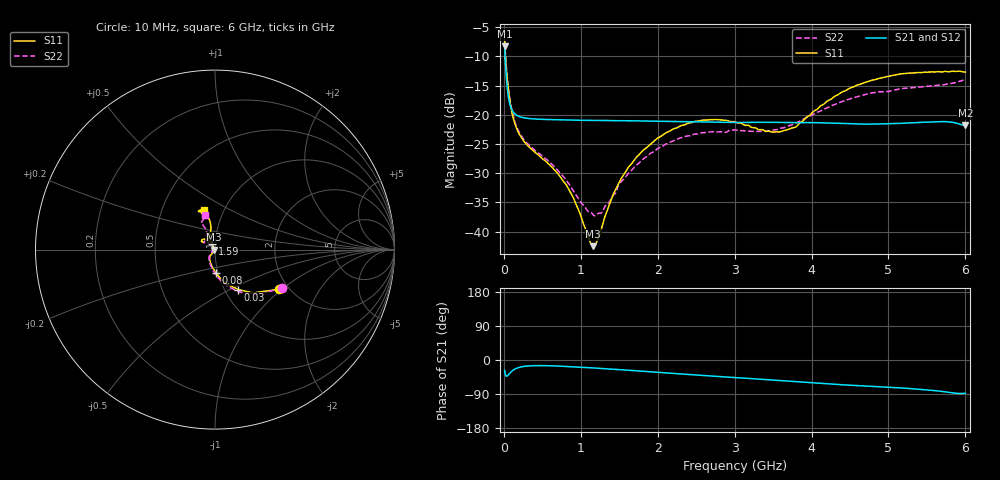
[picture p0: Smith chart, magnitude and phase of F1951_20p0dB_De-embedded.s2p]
! Integrated Device Technology
! Corporate Headquarters
! 6024 Silver Creek Valley Road
! San Jose, CA 95138  USA
! Phone:  1-408-284-8200
! Toll Free:  1-800-223-1366
! Webpage:  http://www.idt.com/
! Timing and RF Division
! 515 Groton Road, Suite 102
! Westford, MA 01886-6024
! Device:  F1951
! Description: 6-bit 0.5 dB Digital Step Attenuator
! Frequency:  100.0 -  4000.00 MHz
! Package:  4x4 mm Thin QFN Plastic Package: 24 pin
! Ports:  2 RF, 6 DC
!  Pin  1  = NC
!  Pin  2  = RF1  =  Port 1
!  Pin  3  = GND
!  Pin  4  = NC
!  Pin  5  = Serial Data Out (SDO)
!  Pin  6  = NC
!  Pin  7  = Reset Bar ( RSTb)
!  Pin  8  = Clock (CLK)
!  Pin  9  = Chip Select Bar (CSb)
!  Pin 10  = NC
!  Pin 11  = Serial Data In (SDI)
!  Pin 12  = NC
!  Pin 13  = NC
!  Pin 14  = VDD
!  Pin 15  = NC
!  Pin 16  = GND
!  Pin 17  = RF2  =  Port 2
!  Pin 18  = NC
!  Pin 19  = GND
!  Pin 20  = GND
!  Pin 21  = GND
!  Pin 22  = GND
!  Pin 23  = GND
!  Pin 24  = GND
! State:  40
! Atten State:  20.0 dB
! Voltage:  +3.30 Volts
! Current:  0.475 mA
! Data:  The device was measured on a F195X evaluation board which has
!  individual transmission lines to the RF pins.  Data was collected
!  de-embedded using a Automatic Fixture Removal [AFR] (Keysight Technologies).
!  The reference plane is the edge of the package pin.
! Misc:  Lot Code  1225BCA
!  Action Tracker AT0399
! Date Measured:  2018-09-13
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# GHz S dB R 50
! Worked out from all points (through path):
!   600 points, 10 MHz to 6 GHz, reference 50 ohm
!   highest |S21| = -8.32 dB at 10 MHz (marker M1); lowest = -21.8 dB at 6 GHz (marker M2)
!   group delay of S21, straight-line fit = 34.6 ps
!   lowest |S11| = -42.5 dB at 1.16 GHz (marker M3), VSWR 1.02, Z = 49.3 + j0.032 ohm
!   |S11| at or under -10 dB: 20.61 MHz to end of sweep
!   |S22| runs from -37.3 to -7.3 dB; largest |S21 - S12| = 0.00023
!   S11 on the Smith chart (normalised r, x): 10 MHz: 1.78, -0.95; 30 MHz: 1.16, -0.55; 80 MHz: 0.98, -0.26; 1.59 GHz: 0.97, +0.06; 6 GHz: 0.80, +0.38
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0.01  -7.55 -31.8  -8.32 -27.2  -8.33 -27.2  -7.30 -30.0
0.03  -11.78 -59.8  -13.09 -42.5  -13.09 -42.6  -11.26 -59.8
0.05  -14.72 -74.5  -16.06 -41.3  -16.06 -41.3  -14.27 -75.5
0.08  -17.80 -88.2  -18.29 -34.3  -18.29 -34.3  -17.41 -89.8
0.15  -21.77 -106.6  -19.94 -23.4  -19.94 -23.4  -21.44 -108.3
0.25  -24.34 -119.1  -20.50 -17.3  -20.50 -17.3  -24.07 -121.8
0.72  -30.37 -126.2  -20.86 -16.2  -20.86 -16.2  -29.78 -135.8
0.88  -33.59 -127.9  -20.91 -17.8  -20.91 -17.9  -32.51 -140.2
1.01  -37.66 -135.8  -20.95 -19.3  -20.95 -19.3  -35.13 -148.4
1.16  -42.48 177.5  -20.97 -21.0  -20.97 -20.9  -37.10 -172.2
1.27  -39.47 132.6  -20.98 -22.4  -20.98 -22.3  -36.78 164.5
1.42  -33.68 116.7  -21.01 -24.4  -21.00 -24.4  -33.77 143.4
1.59  -29.60 115.0  -21.03 -26.6  -21.03 -26.7  -30.49 133.7
2.01  -23.91 125.1  -21.11 -32.7  -21.11 -32.6  -25.69 134.9
2.49  -21.11 138.9  -21.21 -39.4  -21.21 -39.4  -23.30 142.7
3.01  -21.24 149.3  -21.31 -46.5  -21.31 -46.5  -22.60 146.5
3.58  -22.95 128.8  -21.29 -54.2  -21.30 -54.2  -22.39 129.3
3.79  -22.13 112.8  -21.35 -57.2  -21.35 -57.1  -21.41 122.2
4.01  -19.63 103.4  -21.35 -60.2  -21.35 -60.1  -20.04 116.7
4.49  -15.49 100.5  -21.52 -66.4  -21.52 -66.4  -17.32 115.0
5.01  -13.42 108.7  -21.53 -71.7  -21.53 -71.7  -16.00 117.6
6  -12.70 105.8  -21.83 -87.8  -21.83 -87.8  -13.95 106.7
